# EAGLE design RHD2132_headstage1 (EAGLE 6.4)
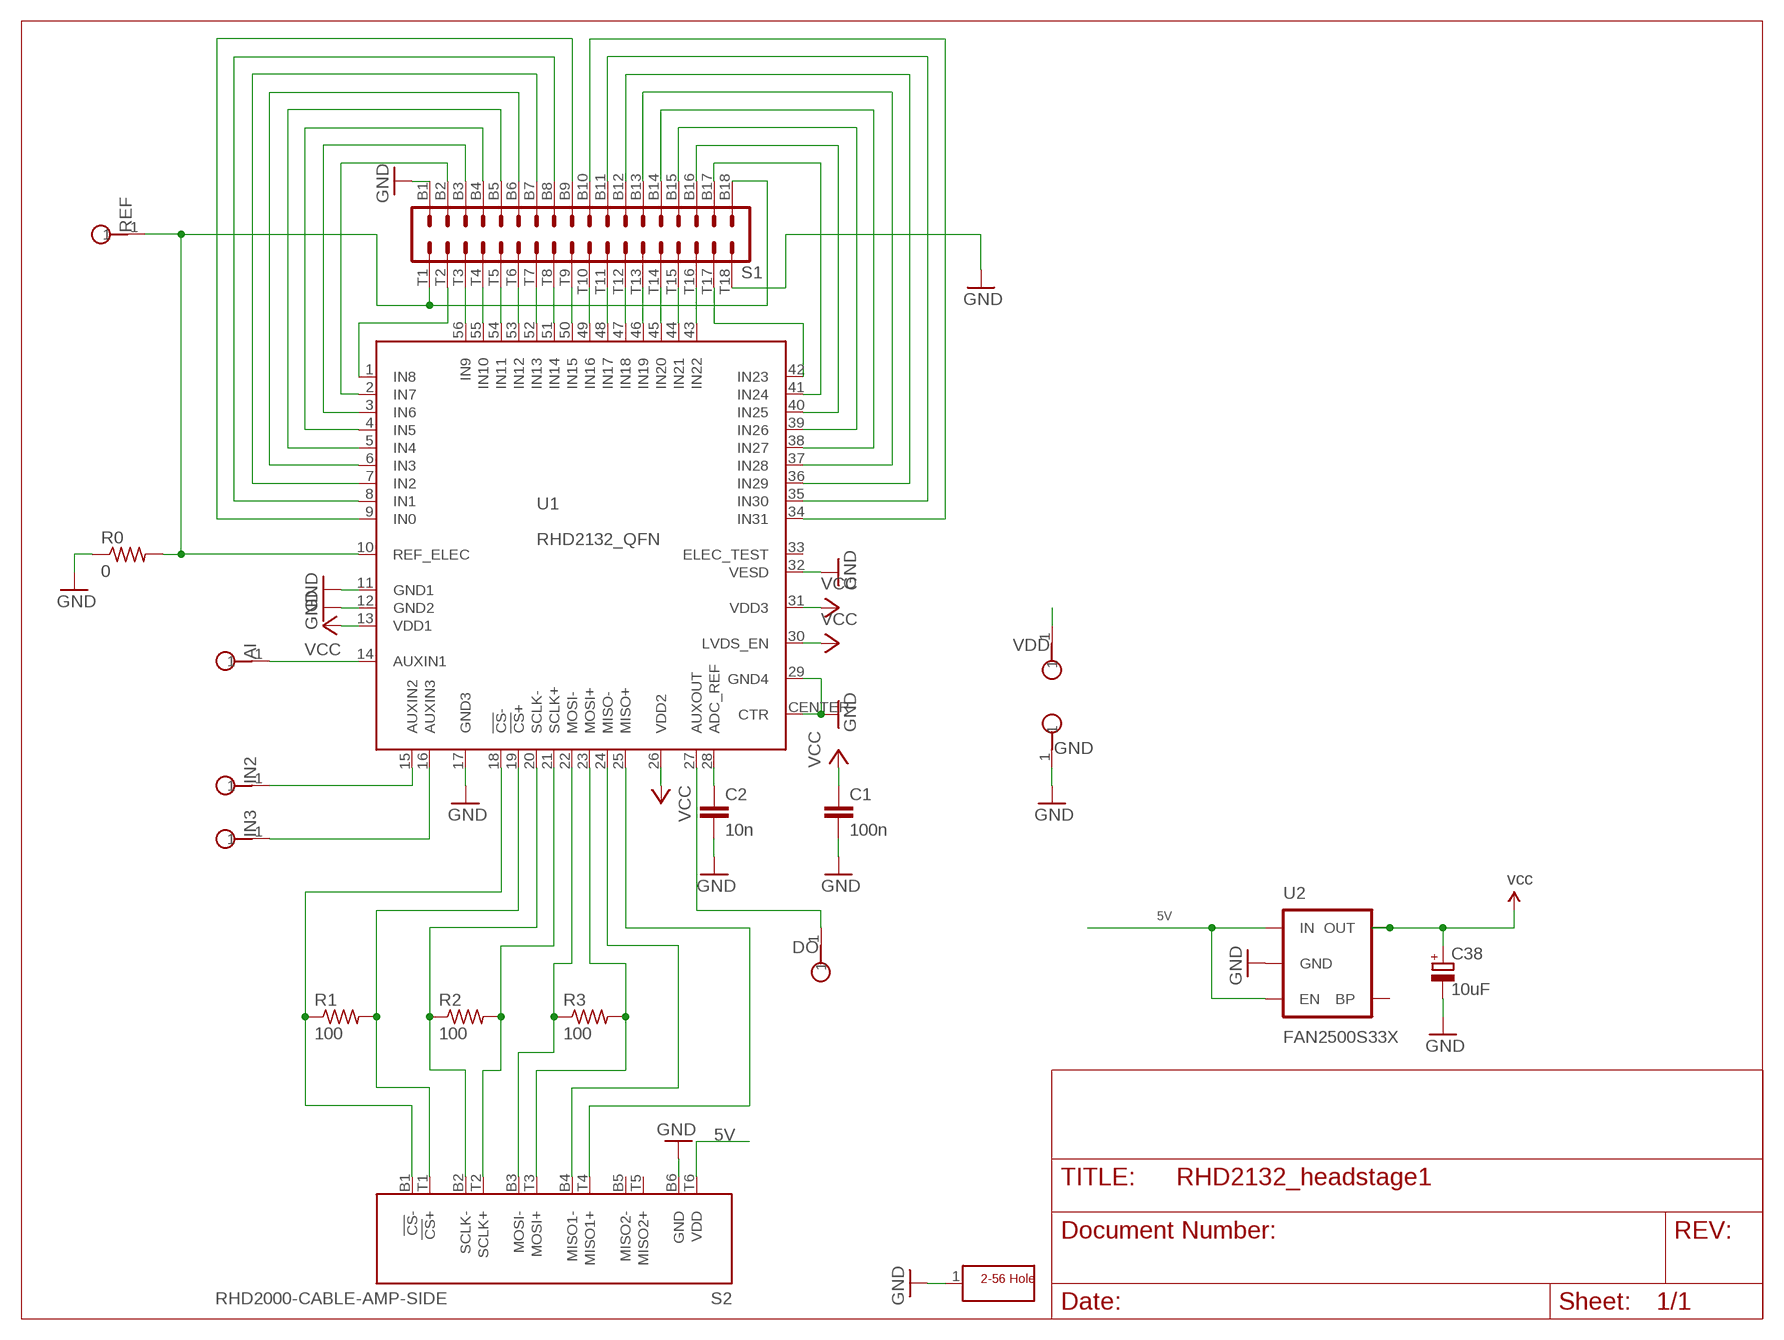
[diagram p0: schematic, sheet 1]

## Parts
AI  TESTPOINT_SMALL  [TESTPOINT_SMALL]
C1  100n  C_0402  [0402]
C2  10n  C_0402  [0402]
C38  10uF  CPOL-EUR/2012-12R  [R/2012-12R]
DO  TESTPOINT_SMALL  [TESTPOINT_SMALL]
GND  TESTPOINT_SMALL  [TESTPOINT_SMALL]
H1  SCREW_HOLE_2-56  [SCREW_HOLE_2-56]
IN2  TESTPOINT_SMALL  [TESTPOINT_SMALL]
IN3  TESTPOINT_SMALL  [TESTPOINT_SMALL]
R0  0  R_0402  [0402]
R1  100  R_0402  [0402]
R2  100  R_0402  [0402]
R3  100  R_0402  [0402]
REF  TESTPOINT_SMALL  [TESTPOINT_SMALL]
S1  OMNETICS_A79025  [OMNETICS_A79025]
S2  RHD2000-CABLE-AMP-SIDE  [OMNETICS_PZN-12-AA]
U1  RHD2132_QFN  [QFN56_8_X_8_LARGE]
U2  FAN2500S33X  V_REG_LDOSMD  [SOT23-5$2]
VDD  TESTPOINT_SMALL  [TESTPOINT_SMALL]

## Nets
5V: S2.T6(VDD) U2.1(IN) U2.3(EN)
GND: C1.2 C2.2 C38.- GND.1 H1.1 R0.1 S1.B1 S1.T18 S2.B6(GND) U1.11(GND1) U1.12(GND2) U1.17(GND3) U1.29(GND4) U1.32(VESD) U1.CENTER(CTR) U2.2(GND)
N$1: R0.2 REF.1 S1.B18 S1.T1 U1.10(REF_ELEC)
N$2: S1.B3 U1.3(IN6)
N$3: S1.B2 U1.2(IN7)
N$4: S1.B4 U1.4(IN5)
N$5: S1.B5 U1.5(IN4)
N$6: S1.B6 U1.6(IN3)
N$7: S1.B7 U1.7(IN2)
N$8: S1.B8 U1.8(IN1)
N$9: S1.B9 U1.9(IN0)
N$11: R1.1 S2.B1(!CS!-) U1.18(!CS!-)
N$12: S1.B17 U1.41(IN24)
N$13: S1.B16 U1.40(IN25)
N$14: S1.B15 U1.39(IN26)
N$15: S1.B14 U1.38(IN27)
N$16: S1.B13 U1.37(IN28)
N$17: S1.B12 U1.36(IN29)
N$18: S1.B11 U1.35(IN30)
N$19: S1.T9 U1.50(IN15)
N$20: S1.T8 U1.51(IN14)
N$21: S1.T7 U1.52(IN13)
N$22: S1.T3 U1.56(IN9)
N$23: S1.T4 U1.55(IN10)
N$24: S1.T5 U1.54(IN11)
N$25: S1.T6 U1.53(IN12)
N$26: S1.T10 U1.49(IN16)
N$27: S1.T11 U1.48(IN17)
N$28: S1.T12 U1.47(IN18)
N$29: S1.T13 U1.46(IN19)
N$30: S1.T14 U1.45(IN20)
N$31: S1.T15 U1.44(IN21)
N$32: S1.T16 U1.43(IN22)
N$33: S1.T2 U1.1(IN8)
N$34: S1.T17 U1.42(IN23)
N$35: R1.2 S2.T1(!CS!+) U1.19(!CS!+)
N$36: R2.1 S2.B2(SCLK-) U1.20(SCLK-)
N$37: R2.2 S2.T2(SCLK+) U1.21(SCLK+)
N$38: R3.1 S2.B3(MOSI-) U1.22(MOSI-)
N$39: R3.2 S2.T3(MOSI+) U1.23(MOSI+)
N$40: S2.B4(MISO1-) U1.24(MISO-)
N$41: S2.T4(MISO1+) U1.25(MISO+)
N$42: C2.1 U1.28(ADC_REF)
N$43: DO.1 U1.27(AUXOUT)
N$44: AI.1 U1.14(AUXIN1)
N$46: IN2.1 U1.15(AUXIN2)
N$48: IN3.1 U1.16(AUXIN3)
N$49: S1.B10 U1.34(IN31)
VCC: C1.1 C38.+ U1.13(VDD1) U1.26(VDD2) U1.30(LVDS_EN) U1.31(VDD3) U2.5(OUT) VDD.1 ; supply symbol labelled vcc
Unconnected: S2.B5(MISO2-) S2.T5(MISO2+) U1.33(ELEC_TEST) U2.4(BP)

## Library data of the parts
AI DO GND IN2 IN3 REF VDD = RHD2000_eval_board:TESTPOINT: PCB Test Point
C1 C2 = RHD2000_eval_board:C: Capacitor
C38 = resistor:CPOL-EU: POLARIZED CAPACITOR, European symbol
H1 = RHD2000_eval_board:SCREW_HOLE_2-56: Mounting hole
R0 R1-R3 = RHD2000_eval_board:R: Resistor
S1 = RHD2000:OMNETICS_A79025
S2 = RHD2000:RHD2000-CABLE-AMP-SIDE
U1 = RHD2000:RHD2132
U2 = SparkFun:V_REG_LDO: Voltage Regulator LDO Standard 150mA LDO voltage regulator in SOT-23 layout. Micrel part MIC5205. BP (by-pass) pin is used to lower output noise with 470pF cap.

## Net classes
1 thick: width 1.016 mm
2 power: width 0.61 mm

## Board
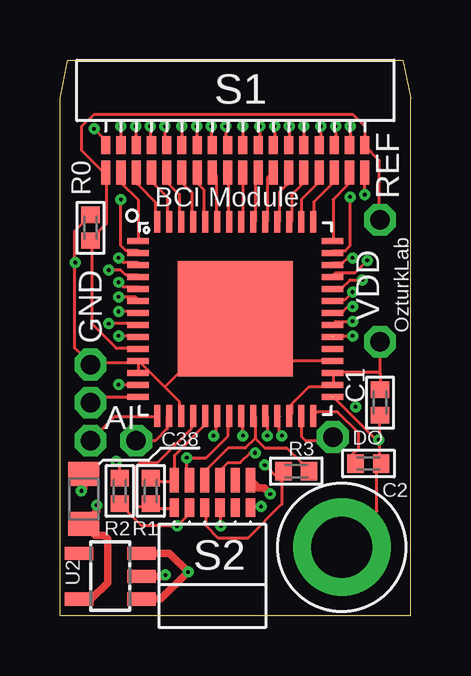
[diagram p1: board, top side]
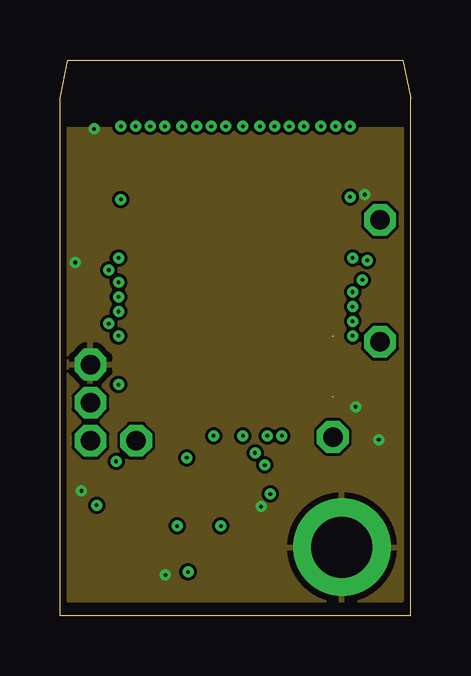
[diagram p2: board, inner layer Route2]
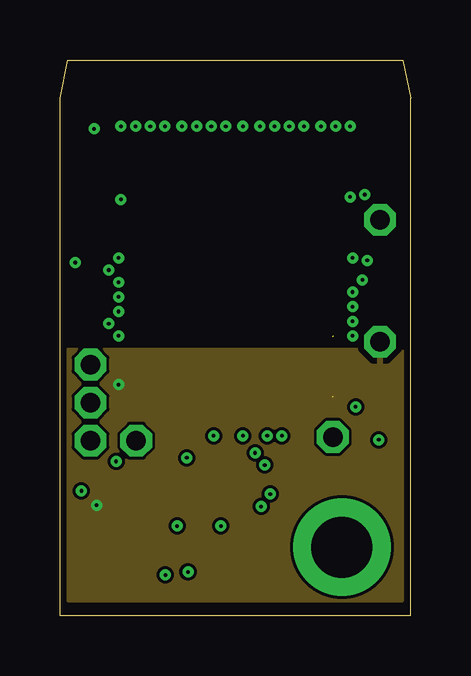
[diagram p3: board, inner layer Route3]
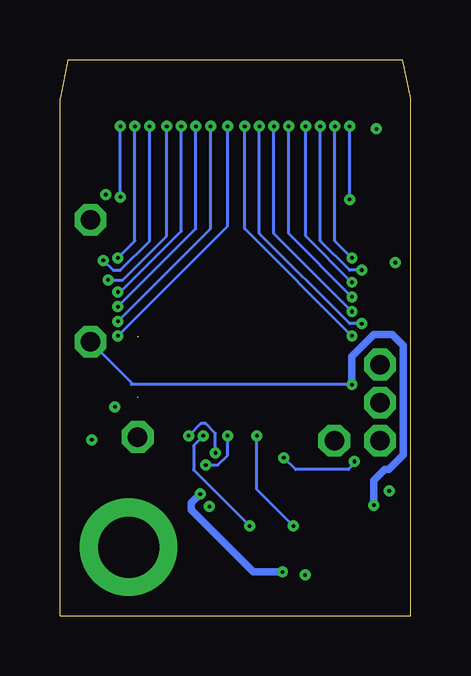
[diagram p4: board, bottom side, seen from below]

Size 14.61 x 23.18 mm. Coordinates in mm from the lower left corner, seen from the top.
Outline: 0,0 0,21.59 0.32,23.18 14.29,23.18 14.61,21.59 14.61,0 0,0
Copper layers (1*2+3*16): Top 0.035mm / dielectric 1.5mm / Route2 0.035mm / dielectric 0.15mm / Route3 0.035mm / dielectric 0.2mm / Bottom 0.035mm
Design rules "default *": minimum track width 5mil, minimum drill 6mil, track to track 5mil, track to pad 5mil, pad to pad 5mil, via to via 5mil, smd to smd 0mil, copper to edge 5mil, drill to drill 5mil, minimum pad ring 10mil, minimum via ring 6mil, stop-mask expansion 4mil, vias tented up to drill 0mil, thermal gap 10mil

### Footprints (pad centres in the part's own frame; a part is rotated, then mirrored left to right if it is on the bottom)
TESTPOINT_SMALL = drill 0.813 octagon: 1 0,0
0402 = smd 0.686 x 0.762: 1 -0.533,0; 2 0.533,0
R/2012-12R = smd 1 x 1.3: + 1.048,0; - -1.048,0
SCREW_HOLE_2-56 = drill 2.54 pad 4.064: 1 0,0
OMNETICS_A79025 = smd 0.381 x 0.762: B1 -5.397,-1.016; B2 -4.763,-1.016; B3 -4.128,-1.016; B4 -3.493,-1.016; B5 -2.857,-1.016; B6 -2.223,-1.016; B7 -1.587,-1.016; B8 -0.953,-1.016; B9 -0.318,-1.016; B10 0.318,-1.016; B11 0.953,-1.016; B12 1.587,-1.016; B13 2.223,-1.016; B14 2.857,-1.016; B15 3.493,-1.016; B16 4.128,-1.016; B17 4.763,-1.016; B18 5.397,-1.016 | smd 0.381 x 1.016: T1 -5.397,-2.159; T2 -4.763,-2.159; T3 -4.128,-2.159; T4 -3.493,-2.159; T5 -2.857,-2.159; T6 -2.223,-2.159; T7 -1.587,-2.159; T8 -0.953,-2.159; T9 -0.318,-2.159; T10 0.318,-2.159; T11 0.953,-2.159; T12 1.587,-2.159; T13 2.223,-2.159; T14 2.857,-2.159; T15 3.493,-2.159; T16 4.128,-2.159; T17 4.763,-2.159; T18 5.397,-2.159
OMNETICS_PZN-12-AA = smd 0.381 x 0.762: B1 1.587,-1.016; B2 0.953,-1.016; B3 0.318,-1.016; B4 -0.318,-1.016; B5 -0.953,-1.016; B6 -1.587,-1.016 | smd 0.381 x 1.016: T1 1.587,-2.159; T2 0.953,-2.159; T3 0.318,-2.159; T4 -0.318,-2.159; T5 -0.953,-2.159; T6 -1.587,-2.159
QFN56_8_X_8_LARGE = smd 0.9 x 0.25: 1 -4.05,3.25; 2 -4.05,2.75; 3 -4.05,2.25; 4 -4.05,1.75; 5 -4.05,1.25; 6 -4.05,0.75; 7 -4.05,0.25; 8 -4.05,-0.25; 9 -4.05,-0.75; 10 -4.05,-1.25; 11 -4.05,-1.75; 12 -4.05,-2.25; 13 -4.05,-2.75; 14 -4.05,-3.25; 29 4.05,-3.25; 30 4.05,-2.75; 31 4.05,-2.25; 32 4.05,-1.75; 33 4.05,-1.25; 34 4.05,-0.75; 35 4.05,-0.25; 36 4.05,0.25; 37 4.05,0.75; 38 4.05,1.25; 39 4.05,1.75; 40 4.05,2.25; 41 4.05,2.75; 42 4.05,3.25 | smd 0.25 x 0.9: 15 -3.25,-4.05; 16 -2.75,-4.05; 17 -2.25,-4.05; 18 -1.75,-4.05; 19 -1.25,-4.05; 20 -0.75,-4.05; 21 -0.25,-4.05; 22 0.25,-4.05; 23 0.75,-4.05; 24 1.25,-4.05; 25 1.75,-4.05; 26 2.25,-4.05; 27 2.75,-4.05; 28 3.25,-4.05; 43 3.25,4.05; 44 2.75,4.05; 45 2.25,4.05; 46 1.75,4.05; 47 1.25,4.05; 48 0.75,4.05; 49 0.25,4.05; 50 -0.25,4.05; 51 -0.75,4.05; 52 -1.25,4.05; 53 -1.75,4.05; 54 -2.25,4.05; 55 -2.75,4.05; 56 -3.25,4.05 | smd 4.8 x 4.8: CENTER 0,0
SOT23-5$2 = smd 0.55 x 1.2: 1 -0.95,-1.3; 2 0,-1.3; 3 0.95,-1.3; 4 0.95,1.3; 5 -0.95,1.3

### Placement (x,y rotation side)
AI  1.27,8.89 90 top
C1  13.34,8.89 270 top
C2  12.85,6.35 0 top
C38  0.99,4.88 270 top
DO  11.37,7.45 0 top
GND  1.27,10.48 0 top
H1  11.75,2.86 0 top
IN2  1.27,7.3 90 top
IN3  3.17,7.3 0 top
R0  1.27,16.18 270 top
R1  3.78,5.21 90 top
R2  2.49,5.21 90 top
R3  9.84,6.03 0 top
REF  13.34,16.51 90 top
S1  7.3,20.64 0 top
S2  6.35,3.49 180 top
U1  7.3,12.38 0 top
U2  2.1,1.65 90 top
VDD  13.34,11.43 0 top

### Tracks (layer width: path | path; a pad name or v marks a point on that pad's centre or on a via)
5V  (via drill 0.15)
  Top 0.305: S2.T6 8.26,5.33 8.51,5.33 v8.76,5.08 | U2.3 4.56,2.6 v5.33,1.83 4.21,0.7 U2.1
  Bottom 0.305: v8.76,5.08 9.14,4.7 9.14,4.42 6.55,1.83 v5.33,1.83
GND  (via drill 0.15)  (1 unrouted)
  Top 0.127: U1.32 11.28,10.65 9.04,10.65 7.32,12.38 U1.CENTER 7.21,12.38 4.37,9.54 | 13.31,7.2 13.31,8.32 C1.2 | 13.31,7.2 13.31,6.39 C2.2 13.21,6.29 13.21,4.36 11.79,2.93 H1.1 | 13.31,7.2 11.38,9.13 | 3.25,10.55 3.25,10.15 U1.12 | 4.37,9.54 3.35,10.55 U1.11 3.25,10.55 | 4.37,9.54 4.98,8.93 4.98,8.42 U1.17 | 7.92,4.56 S2.B6 8.03,4.56 v8.38,4.56 | R0.1 1.22,16.65 0.61,16.04 0.61,11.16 1.22,10.55 GND.1 1.32,10.55 3.25,10.55 | v1.42,20.31 1.83,19.9 1.83,19.7 S1.B1 | v12.7,17.56 S1.T18
  Top 0.305: U2.2 4.34,1.65 v4.39,1.7 | C38.- 0.99,5.31 v0.89,5.21
  other vias: 12.32,8.71 13.28,7.34 0.64,14.73
  pour Route2: 0.32,0.64 14.29,0.64 14.29,20.32 0.32,20.32
N$1
  Top 0.127: REF.1 13.31,16.55 13.31,18.99 12.7,19.6 S1.B18 12.7,20.41 12.19,20.92 1.42,20.92 0.91,20.41 0.91,19.39 1.83,18.48 S1.T1 1.93,18.48 1.93,16.34 1.32,15.73 R0.2 1.32,15.63 1.32,12.18 2.34,11.16 3.25,11.16 U1.10
N$2  (via drill 0.15)
  Top 0.127: v3.15,20.41 3.15,19.7 S1.B3 | v2.44,14.92 2.64,14.72 3.25,14.72 U1.3
  Bottom 0.127: v3.15,20.41 3.15,15.63 v2.44,14.92
N$3  (via drill 0.15)
  Top 0.127: v2.54,20.41 S1.B2 | v2.54,17.36 2.54,15.43 2.74,15.23 3.25,15.23 U1.2
  Bottom 0.127: v2.54,17.36 v2.54,20.41
N$4  (via drill 0.15)
  Top 0.127: v3.76,20.41 3.76,19.7 S1.B4 | v2.03,14.41 2.54,14.41 2.74,14.21 3.25,14.21 U1.4
  Bottom 0.127: v3.76,20.41 3.76,15.63 2.54,14.41 v2.03,14.41
N$5  (via drill 0.15)
  Top 0.127: v4.37,20.41 4.37,19.7 S1.B5 | v2.44,13.91 2.64,13.7 3.25,13.7 U1.5
  Bottom 0.127: v4.37,20.41 4.37,15.84 v2.44,13.91
N$6  (via drill 0.15)
  Top 0.127: v5.08,20.41 S1.B6 | v2.44,13.3 3.15,13.3 3.25,13.2 U1.6
  Bottom 0.127: v5.08,20.41 5.08,15.94 v2.44,13.3
N$7  (via drill 0.15)
  Top 0.127: v5.69,20.41 5.69,19.7 S1.B7 | v2.44,12.69 3.25,12.69 U1.7
  Bottom 0.127: v5.69,20.41 5.69,15.94 v2.44,12.69
N$8  (via drill 0.15)
  Top 0.127: v6.3,20.41 6.3,19.7 S1.B8 | v2.03,12.18 3.25,12.18 U1.8
  Bottom 0.127: v6.3,20.41 6.3,15.94 2.54,12.18 v2.03,12.18
N$9  (via drill 0.15)
  Top 0.127: v6.91,20.41 6.91,19.7 S1.B9 | v2.44,11.67 3.25,11.67 U1.9
  Bottom 0.127: v6.91,20.41 6.91,16.14 v2.44,11.67
N$11
  Top 0.127: S2.B1 4.67,4.46 3.85,4.46 R1.1 3.52,4.56 3.15,4.56 3.15,6.2 3.35,6.4 4.08,6.4 | 4.06,6.39 4.08,6.4 | 4.08,6.4 5.49,7.81 5.49,8.32 U1.18
N$12  (via drill 0.15)
  Top 0.127: v12.09,20.41 12.09,19.7 S1.B17 | v12.09,17.46 12.09,15.43 11.89,15.23 11.38,15.23 U1.41
  Bottom 0.127: v12.09,17.46 v12.09,20.41
N$13  (via drill 0.15)
  Top 0.127: v11.48,20.41 11.48,19.7 S1.B16 | v12.19,14.92 11.99,14.92 11.79,14.72 11.38,14.72 U1.40
  Bottom 0.127: v11.48,20.41 11.48,15.63 v12.19,14.92
N$14  (via drill 0.15)
  Top 0.127: v10.87,20.41 10.87,19.7 S1.B15 | v12.8,14.82 12.29,14.31 11.48,14.31 11.38,14.21 U1.39
  Bottom 0.127: v10.87,20.41 10.87,15.63 12.09,14.41 12.39,14.41 v12.8,14.82
N$15  (via drill 0.15)
  Top 0.127: v10.16,20.41 S1.B14 | v12.6,14.01 12.09,14.01 11.79,13.7 11.38,13.7 U1.38
  Bottom 0.127: v10.16,20.41 10.16,15.84 11.99,14.01 v12.6,14.01
N$16  (via drill 0.15)
  Top 0.127: v9.55,20.41 9.55,19.7 S1.B13 | v12.19,13.5 11.89,13.2 11.38,13.2 U1.37
  Bottom 0.127: v9.55,20.41 9.55,16.04 12.09,13.5 v12.19,13.5
N$17  (via drill 0.15)
  Top 0.127: v8.94,20.41 8.94,19.7 S1.B12 | v12.19,12.89 11.99,12.89 11.79,12.69 11.38,12.69 U1.36
  Bottom 0.127: v8.94,20.41 8.94,16.14 v12.19,12.89
N$18  (via drill 0.15)
  Top 0.127: v8.33,20.41 8.33,19.7 S1.B11 | v12.19,12.28 11.48,12.28 11.38,12.18 U1.35
  Bottom 0.127: v8.33,20.41 8.33,16.14 v12.19,12.28
N$19
  Top 0.127: U1.50 7.01,16.45 7.01,18.48 S1.T9
N$20
  Top 0.127: U1.51 6.5,16.45 6.5,18.38 6.4,18.48 S1.T8
N$21
  Top 0.127: U1.52 5.99,16.45 5.99,17.77 5.79,17.97 5.79,18.48 S1.T7
N$22
  Top 0.127: U1.56 3.96,16.45 3.96,17.26 3.25,17.97 3.25,18.48 S1.T3
N$23
  Top 0.127: U1.55 4.47,16.45 4.47,17.46 3.86,18.07 3.86,18.48 S1.T4
N$24
  Top 0.127: U1.54 4.98,16.45 4.98,17.56 4.47,18.07 4.47,18.48 S1.T5
N$25
  Top 0.127: S1.T6 5.08,18.07 5.49,17.67 5.49,16.45 U1.53
N$26
  Top 0.127: S1.T10 7.62,16.45 U1.49
N$27
  Top 0.127: U1.48 8.13,16.45 8.13,18.38 8.23,18.48 S1.T11
N$28
  Top 0.127: U1.47 8.64,16.45 8.64,18.27 8.84,18.48 S1.T12
N$29
  Top 0.127: U1.46 9.14,16.45 9.14,17.67 9.45,17.97 9.45,18.48 S1.T13
N$30
  Top 0.127: S1.T14 10.16,18.07 9.65,17.56 9.65,16.45 U1.45
N$31
  Top 0.127: U1.44 10.06,16.45 10.06,17.36 10.77,18.07 10.77,18.48 S1.T15
N$32
  Top 0.127: U1.43 10.57,16.45 10.57,17.26 11.38,18.07 11.38,18.48 S1.T16
N$33
  Top 0.127: S1.T2 2.54,18.07 3.25,17.36 U1.1
N$34
  Top 0.127: U1.42 11.38,15.63 11.38,17.36 11.99,17.97 11.99,18.48 S1.T17
N$35
  Top 0.127: U1.19 5.99,8.32 5.99,7.91 4.78,6.69 4.78,5.68 S2.T1 4.67,5.58 3.8,5.58 R1.2
N$36  (via drill 0.15)
  Top 0.127: S2.B2 5.38,4.46 5.38,4.25 v4.88,3.75 3.42,3.75 R2.1 | v6.4,7.51 6.5,7.61 6.5,8.32 U1.20
  Bottom 0.127: v6.4,7.51 6.4,5.27 v4.88,3.75
N$37  (via drill 0.15)
  Top 0.127: S2.T2 5.38,5.68 5.28,5.78 v5.28,6.59 6.1,6.59 7.01,7.51 7.01,8.32 U1.21 | R2.2 2.49,6.29 v2.34,6.44
  Bottom 0.127: v2.34,6.44 2.34,6.35 2.59,6.1 4.79,6.1 v5.28,6.59
N$38  (via drill 0.15)
  Top 0.127: 9.25,5.58 9.25,5.98 R3.1 | 9.25,5.58 9.25,4.66 7.82,3.24 6.6,3.24 6.1,3.75 6.1,4.46 S2.B3 | v7.62,7.51 7.62,8.32 U1.22 | 9.25,5.58 v8.53,6.29
  Bottom 0.127: v7.62,7.51 7.62,6.69 8.03,6.29 v8.53,6.29
N$39
  Top 0.127: 8.13,7.4 8.53,7 9.45,7 10.36,6.08 R3.2 | 8.13,7.4 8.13,8.32 U1.23 | 8.13,7.4 7.72,7 7.01,7 6.1,6.08 6.1,5.68 S2.T3
N$40  (via drill 0.15)
  Top 0.127: v6.71,3.75 6.71,4.46 S2.B4 | v8.64,7.51 8.64,8.32 U1.24
  Bottom 0.127: v6.71,3.75 9.04,6.08 9.04,7.1 v8.64,7.51
N$41  (via drill 0.15)
  Top 0.127: v9.25,7.51 9.14,7.61 9.14,8.32 U1.25 | v8.13,6.79 7.92,6.79 7.52,6.39 7.01,6.39 6.71,6.08 6.71,5.68 S2.T4
  Bottom 0.127: v9.25,7.51 8.74,8.01 8.53,8.01 8.13,7.61 v8.13,6.79
N$42
  Top 0.127: C2.1 12.17,6.71 12.45,6.99 12.45,7.62 11.56,8.51 10.73,8.51 U1.28
N$43
  Top 0.127: U1.27 10.05,7.47 10.21,7.32 11.23,7.32 DO.1
N$44
  Top 0.127: AI.1 1.83,9.13 U1.14
N$46
  Top 0.127: U1.15 3.96,8.32 2.29,8.32 IN2.1
N$48
  Top 0.127: U1.16 4.47,8.32 4.47,7.81 3.96,7.3 IN3.1
N$49  (via drill 0.15)  (1 unrouted)
  Top 0.127: v7.62,20.41 S1.B10 | 11.38,11.67 v12.19,11.67
  Bottom 0.127: v7.62,20.41 7.62,16.24 v12.19,11.67
VCC  (via drill 0.15)
  Top 0.127: U1.26 9.65,8.42 9.65,8.83 10.36,9.54 11.28,9.54 U1.30 11.38,9.64 11.38,10.05 U1.31 11.38,10.15 13.31,10.15 | 13.31,9.44 C1.1 13.34,10.12 13.31,10.15 | v2.44,9.64 U1.13 | 13.31,10.15 13.34,10.17 VDD.1
  Top 0.305: U2.5 1.31,0.7 1.98,1.37 1.98,3.2 1.83,3.35 1.47,3.35 C38.+ 1.52,4.36 v1.52,4.61
  Bottom 0.127: v2.44,9.64 11.62,9.64 11.62,9.72 VDD.1
  Bottom 0.305: v1.52,4.61 1.52,5.64 1.07,6.1 0.91,6.1 0.3,6.71 0.3,11.28 0.76,11.73 1.52,11.73 2.44,10.82 2.44,9.75
  pour Route3: 0.32,0.64 14.29,0.64 14.29,11.11 0.32,11.11

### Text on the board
tPlace: BCI Module | OzturkLab

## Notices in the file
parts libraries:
SparkFun: Licensing: CC v3.0 Share-Alike You are welcome to use this library for commercial purposes.
